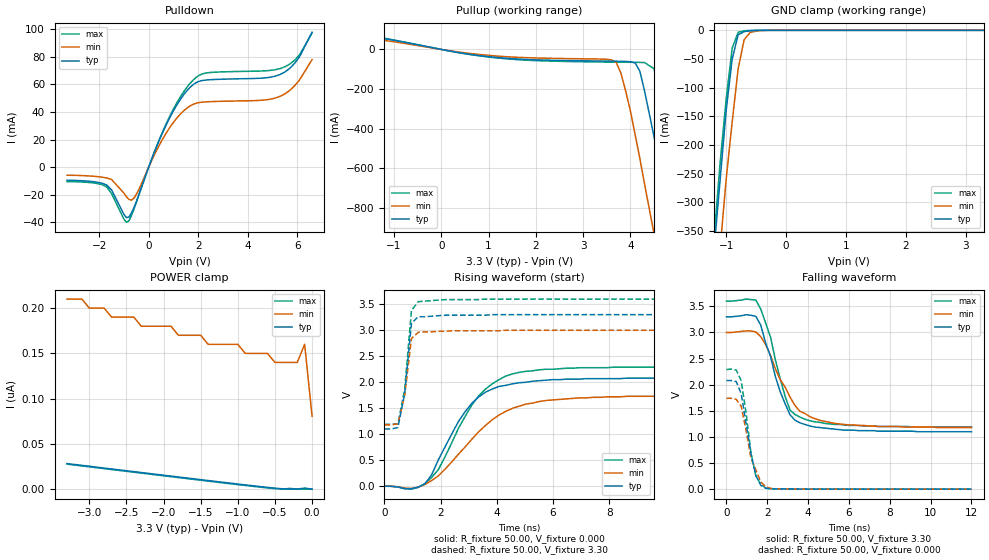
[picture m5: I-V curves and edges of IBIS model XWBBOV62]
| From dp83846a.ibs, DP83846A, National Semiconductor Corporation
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|   Model XWBBOV62
[Model]   XWBBOV62
Model_type   I/O
Polarity   Non-Inverting
Enable   Active-High
Vinl =   0.80V
Vinh =   2.00V
Vmeas =   1.50V
Cref =  20.00pF
Rref = 100.00k
C_comp   5.00pF   5.00pF   5.00pF
[Temperature Range]   25.00   0.14k   0.000
[Voltage Range]   3.30V   3.00V   3.60V
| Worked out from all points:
|   slope of the pulldown table from 0 to 0.495 V, typ, clamps not added: 22.2 ohm
|   slope of the pullup table from 0 to 0.495 V, typ, clamps not added: 24 ohm
|   GND clamp passes 1 mA (typ) near -0.61 V on its own axis
|   rising waveform, R_fixture 50.00, V_fixture 0.000: 20-80 % time 1.41ns typ, 1.96ns min, 1.48ns max; typ from 0 V to 2.08 V
|   rising waveform, R_fixture 50.00, V_fixture 3.30: 20-80 % time 283ps typ, 285ps min, 269ps max; typ from 1.1 V to 3.3 V
|   falling waveform, R_fixture 50.00, V_fixture 3.30: 20-80 % time 1.11ns typ, 1.41ns min, 995ps max; typ from 3.3 V to 1.1 V
|   falling waveform, R_fixture 50.00, V_fixture 0.000: 20-80 % time 561ps typ, 640ps min, 513ps max; typ from 2.08 V to 0 V
[Pulldown]
| voltage   I(typ)   I(min)   I(max)
-3.3V     -9.54mA    -5.89mA    -10.52mA
-1.7V     -12.98mA   -7.9mA     -14.33mA
-1V       -34.44mA   -18.95mA   -37.9mA
-800mV    -36.29mA   -23.47mA   -38.99mA
-500mV    -25.06mA   -19.83mA   -25.59mA
700mV     30.4mA     24.48mA    31.2mA
1.3V      49.68mA    38.87mA    51.57mA
1.8V      59.89mA    45.59mA    63.21mA
2.4V      63.31mA    47.42mA    68.48mA
5.3V      67.13mA    51.27mA    71.44mA
5.9V      75.39mA    59.1mA     77.64mA
6.6V      97.97mA    78.03mA    97.27mA
[Pullup]
| voltage   I(typ)   I(min)   I(max)
-3.3V     5.38mA     4.26mA     6.06mA
-2.5V     91.42mA    11.58mA    99.58mA
-1.9V     81.05mA    64.78mA    84.48mA
3.6V      -59.14mA   -52.56mA   -64.06mA
3.8V      -59.72mA   -120mA     -64.53mA
4.1V      -67.93mA   -430mA     -65.17mA
4.3V      -210mA     -680mA     -66.35mA
4.5V      -440mA     -930mA     -97.26mA
4.9V      -960mA     -1.45A     -550mA
5.1V      -1.22A     -1.71A     -810mA
5.3V      -1.49A     -1.98A     -1.07A
6.6V      -3.25A     -3.72A     -2.83A
[GND_clamp]
| voltage   I(typ)   I(min)   I(max)
-3.3V     -3.19A     -3.26A     -3.16A
-1.2V     -380mA     -500mA     -360mA
-1.1V     -260mA     -380mA     -230mA
-1V       -140mA     -260mA     -120mA
-900mV    -50.3mA    -160mA     -31.38mA
-800mV    -7.8mA     -66.86mA   -3.4mA
-700mV    -2.29mA    -16.45mA   -820uA
-600mV    -810uA     -3.75mA    -150uA
-500mV    -150uA     -1.28mA    -12.72uA
-200mV    -30.88nA   -7.81uA    -690pA
3.3V      76.46pA    140nA      35.95pA
[POWER_clamp]
| voltage   I(typ)   I(min)   I(max)
-3.3V     28.3nA     210nA      27.68nA
-2.8V     23.34nA    200nA      22.72nA
-2.7V     22.35nA    190nA      21.73nA
-2.4V     19.39nA    190nA      18.76nA
-2.3V     18.4nA     180nA      17.77nA
-1.5V     10.54nA    170nA      9.91nA
-1.4V     9.56nA     160nA      8.93nA
-1V       5.7nA      160nA      5.07nA
-500mV    1.16nA     140nA      630pA
-200mV    99.2pA     140nA      140pA
-100mV    1.26nA     160nA      43.71pA
0V        76.46pA    80.59nA    39.37pA
[Ramp]
| variable   typ   min   max
dV/dt_r   1.90/0.55n   1.71/0.75n   2.07/0.54n
dV/dt_f   1.90/0.52n   1.71/0.66n   2.07/0.52n
R_load = 0.50k
[Rising Waveform]
R_fixture = 50.00
V_fixture = 0.000
V_fixture_min = 0.000
V_fixture_max = 0.000
| time   V(typ)   V(min)   V(max)
0s        230uV      210uV      260uV
960ps     -47.54mV   -43.57mV   -56.64mV
1.44ns    46.57mV    32.31mV    49.65mV
1.92ns    510mV      200mV      320mV
2.64ns    1.25V      620mV      1.12V
3.12ns    1.6V       910mV      1.57V
3.6ns     1.81V      1.17V      1.87V
4.32ns    1.94V      1.44V      2.12V
6.96ns    2.06V      1.7V       2.28V
12ns      2.08V      1.74V      2.29V
[Rising Waveform]
R_fixture = 50.00
V_fixture = 3.30
V_fixture_min = 3.00
V_fixture_max = 3.60
| time   V(typ)   V(min)   V(max)
0s        1.1V       1.18V      1.19V
240ps     1.1V       1.18V      1.19V
480ps     1.13V      1.2V       1.2V
720ps     1.79V      1.75V      1.87V
960ps     3.13V      2.84V      3.38V
1.2ns     3.26V      2.96V      3.55V
2.16ns    3.29V      2.98V      3.59V
3.6ns     3.29V      2.99V      3.6V
3.84ns    3.3V       2.99V      3.6V
12ns      3.3V       3V         3.6V
[Falling Waveform]
R_fixture = 50.00
V_fixture = 3.30
V_fixture_min = 3.00
V_fixture_max = 3.60
| time   V(typ)   V(min)   V(max)
0s        3.3V       3V         3.6V
1.44ns    3.31V      3.01V      3.62V
1.68ns    3.14V      2.92V      3.45V
2.16ns    2.54V      2.56V      2.91V
2.64ns    1.86V      2.09V      2.1V
3.12ns    1.42V      1.76V      1.51V
3.6ns     1.27V      1.49V      1.38V
4.56ns    1.18V      1.32V      1.28V
6ns       1.13V      1.23V      1.22V
12ns      1.1V       1.18V      1.19V
[Falling Waveform]
R_fixture = 50.00
V_fixture = 0.000
V_fixture_min = 0.000
V_fixture_max = 0.000
| time   V(typ)   V(min)   V(max)
0s        2.08V      1.74V      2.29V
480ps     2.06V      1.72V      2.28V
720ps     1.83V      1.59V      2.08V
960ps     1.26V      1.13V      1.46V
1.2ns     680mV      590mV      700mV
1.44ns    260mV      370mV      250mV
1.68ns    73.32mV    140mV      96.1mV
1.92ns    17.04mV    46.59mV    21.75mV
2.88ns    3.9mV      4.05mV     4.47mV
12ns      28.2uV     66.96uV    37.61uV
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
